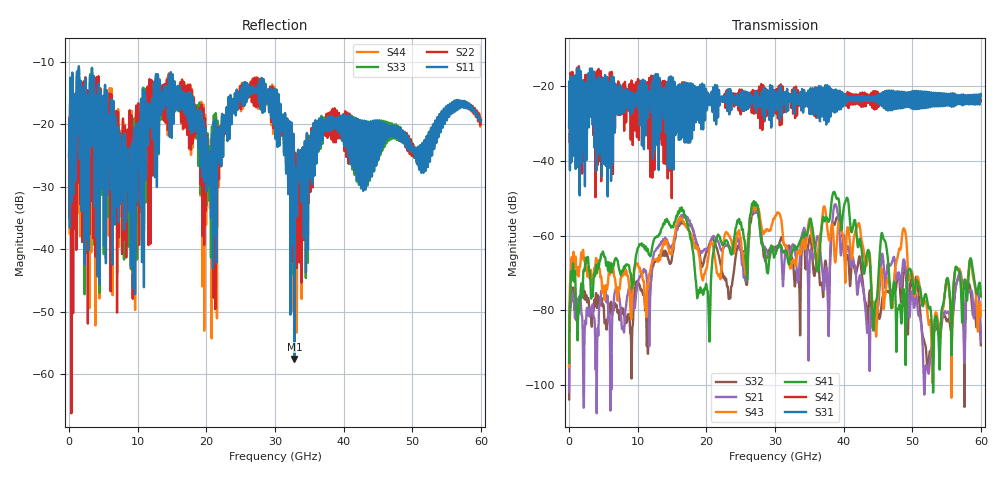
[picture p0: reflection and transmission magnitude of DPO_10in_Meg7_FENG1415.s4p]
! Tyco Electronics Strada Whisper System
! FEXT_G1415_G1112
!! SYSTEM DESCRIPTION: Daughtercard-Footprint-Connector-Footprint-Daughtercard
!! PCB DESCRIPTION: DC: 140mil, Megtron7N, upper layer route, 15mil stub, 6-6-6mil 10" traces
!! CONNECTOR DESCRIPTION: Next-Gen STRADA Whisper Direct-Plug Orthogonal Connector
!! MODEL DESCRIPTION: Tyco Electronics System 4-port S-parameter
!! MODEL STATUS: Developmental
!! MODEL GEOMETRY: Channel Model
!! MODEL FREQUENCY RANGE: DC to 60 GHz in 10 MHz frequency steps
!! MODEL EDGE RATE LIMITATION: 8.3 ps (Using conservative 0.5/Fmax rule of thumb)
!! TIME-DOMAIN TRANSFORM CAUTIONS:
!! 1.) Do not simulate transient edge rates faster than the number listed above.  Edge rates faster than this number
!!  contain significant spectral content at frequencies above the model's highest frequency.
!! 2.) Even when simulating edge rates that are slower than the number listed above, be aware that the best time
!!  resolution possible with a direct iFFT is (1 / 2Fmax).  As a result, time resolution is typically not adequate
!!  for most time-domain simulations unless tricks such as windowing are used to minimize leakage and aliasing.
!! 3.) Because the model has a uniform frequency step, a direct iFFT will result in an impulse that that has a time
!!  length given by either (1 / Fstep) or (1 / 2Fstep), depending on the transform being used.  Care has been taken
!!  in selecting the frequency step to ensure a settled impulse response for the model.  Therefore, convolution with
!!  the model's impulse response should present no issues.  However, if directly concatenating s-parameter models
!!  in the frequency domain a user must either interpolate necessary interim frequencies or complete impulse response
!!  zero-padding.  Impulse response zero-padding is more difficult, but more accurate.
!! PORT DEFINITIONS:
!! Port  1  ----->  TX Side	G14  G11  RX Side  <-----  Port  3
!! Port  2  ----->  TX Side	G15  G12  RX Side  <-----  Port  4
! Touchstone data
! Created: 10-Dec-2018 by IdEM R2012 (8.0.5)
# Hz S MA R 50
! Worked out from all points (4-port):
!   6000 points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, 10 MHz to 60 GHz, reference 50 ohm
!   strongest paths, dB at 10 MHz, 15.01 GHz, 30.01 GHz, 45.01 GHz, 60 GHz:
!     S31: -30.8, -24.1, -24.8, -23.5, -22.6
!     S42: -31.1, -23.8, -22.2, -22.9, -23.6
!     S41: -94.1, -57.6, -65.0, -72.8, -76.3
!     S43: -95.3, -63.9, -54.9, -76.6, -81.6
!     S21: -102.0, -62.7, -64.0, -79.2, -88.5
!     S32: -103.9, -65.7, -63.6, -80.5, -89.4
!   lowest |S11| = -57.5 dB at 32.84 GHz (marker M1), VSWR 1.00, Z = 50 - j0.133 ohm
!   |S11| at or under -10 dB: start of sweep to end of sweep
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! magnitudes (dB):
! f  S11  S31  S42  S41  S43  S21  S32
! 10 MHz  -25.4  -30.8  -31.1  -94.1  -95.3  -102.0  -103.9
! 16.39 GHz  -14.9  -20.1  -26.3  -52.5  -55.5  -54.5  -56.3
! 20.35 GHz  -29.2  -24.6  -23.3  -82.4  -64.7  -63.8  -62.9
! 27.17 GHz  -14.3  -21.9  -23.9  -51.2  -52.7  -53.2  -53.3
! 32.84 GHz  -57.5  -25.0  -21.7  -62.8  -67.2  -63.2  -72.6
! 39.14 GHz  -21.1  -21.2  -25.8  -50.2  -58.7  -54.0  -55.1
! 60 GHz  -19.6  -22.6  -23.6  -76.3  -81.6  -88.5  -89.4
